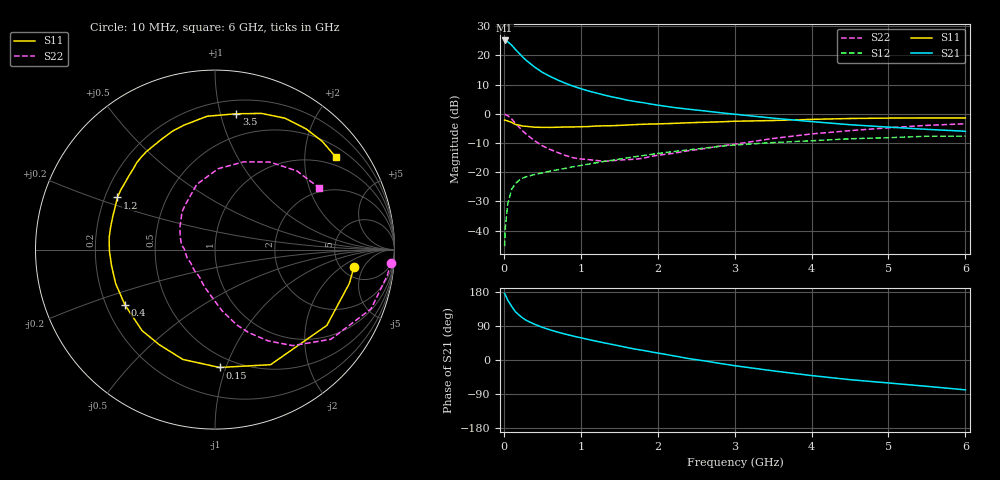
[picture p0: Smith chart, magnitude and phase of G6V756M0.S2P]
! SIEMENS Small Signal Semiconductors
! BFG193
! Si NPN RF Bipolar Junction Transistor in SOT223
! VCE = 0.75 V  IC = 6 mA
! Common Emitter S-Parameters:  August  1996
# GHz  S  MA  R  50
!  f  S11  S21  S12  S22
! GHz  MAG  ANG  MAG  ANG  MAG  ANG  MAG  ANG
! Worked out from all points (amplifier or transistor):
!   36 points, 10 MHz to 6 GHz, reference 50 ohm
!   highest |S21| = 25.1 dB at 10 MHz (marker M1)
!   |S21| within 3 dB of that: start of sweep to 147.9 MHz
!   unconditionally stable (mu >= 1): 978 MHz to 3.691 GHz
!   at 250 MHz: K = 0.40, MSG = 20.7 dB, |S12| = -22.0 dB
!   at 1.4 GHz: K = 1.10, MAG = 8.9 dB, |S12| = -16.0 dB
!   at 6 GHz: K = 0.98, MSG = 0.8 dB, |S12| = -7.7 dB
!   S11 on the Smith chart (normalised r, x): 10 MHz: 6.46, -3.23; 150 MHz: 0.41, -0.95; 400 MHz: 0.28, -0.26; 1.2 GHz: 0.25, +0.24; 3.5 GHz: 0.31, +1.12; 6 GHz: 0.76, +2.78
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0.01  0.7803 -7.2  18.01 175.5  0.0054 88.3  0.9821 -4.2
0.02  0.7717 -14.2  17.98 172.0  0.0113 85.5  0.971 -8.5
0.05  0.7528 -34.1  17.15 158.3  0.0283 73.2  0.93 -20.8
0.1  0.7121 -64.2  15.04 142.0  0.0503 60.5  0.8165 -37.7
0.15  0.6572 -87.8  12.66 127.5  0.0637 50.4  0.6884 -51.0
0.2  0.6377 -106.3  10.81 118.1  0.073 45.0  0.5883 -59.8
0.25  0.614 -120.4  9.236 110.0  0.0795 40.5  0.5 -67.8
0.3  0.6074 -132.0  8.038 103.7  0.0843 38.4  0.4388 -73.7
0.4  0.5888 -148.6  6.313 94.3  0.0911 35.6  0.3439 -83.3
0.5  0.585 -161.2  5.137 86.2  0.097 34.2  0.2834 -90.7
0.6  0.5833 -171.2  4.369 79.6  0.1039 34.4  0.2452 -97.7
0.7  0.5883 -179.1  3.789 73.6  0.1099 34.3  0.217 -105.2
0.9  0.595 167.7  2.974 63.3  0.124 34.2  0.1764 -119.1
1.1  0.6045 156.9  2.455 54.1  0.1371 33.8  0.164 -133.9
1.2  0.6165 151.9  2.271 49.7  0.1446 33.5  0.1585 -141.4
1.6  0.6414 134.9  1.713 33.0  0.1757 29.9  0.1637 -169.3
2.2  0.6837 115.7  1.287 11.3  0.225 21.3  0.2099 157.7
2.8  0.7268 98.4  1.047 -8.7  0.2761 10.2  0.2791 131.3
3.5  0.766 81.1  0.841 -28.6  0.3214 -5.6  0.3777 105.5
4.5  0.8298 61.9  0.649 -51.9  0.373 -24.5  0.514 72.0
5.5  0.8491 45.3  0.541 -69.5  0.4122 -47.2  0.6329 43.8
6  0.848 37.3  0.501 -78.7  0.4126 -60.1  0.6745 30.7
